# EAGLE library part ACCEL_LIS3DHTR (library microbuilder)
LIS3DHTR 3-Axis Accelerometer with I2C/SPI Interface VDD: 1.71-3.6V VDDIO: 1.71-VDD+0.1V Scale: +/-2g, 4g, 8g, 16g with 16--bit data output Temp:: -40°C - 85°C Mouser: 511-LIS3DHTR Digikey: 497-10613-1-ND
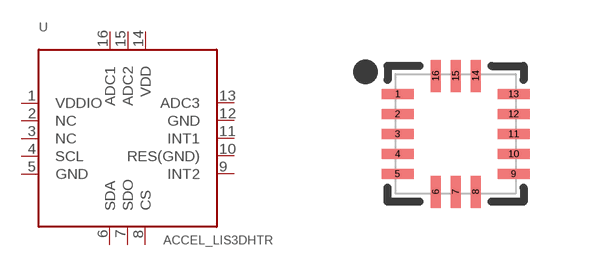
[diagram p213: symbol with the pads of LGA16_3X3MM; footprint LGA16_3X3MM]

Designator prefix U

## ACCEL_LIS3DHTR  [LGA16_3X3MM]
1  VDDIO  sup
2  NC  nc
3  NC  nc
4  SCL
5  GND  sup
6  SDA
7  SDO
8  CS  in
9  INT2  out
10  RES(GND)
11  INT1  out
12  GND  sup
13  ADC3  in
14  VDD  sup
15  ADC2  in
16  ADC1  in

## Footprint LGA16_3X3MM (pad centres in mm)
smd 0.8 x 0.25: 1 -1.45,1; 2 -1.45,0.5; 3 -1.45,0; 4 -1.45,-0.5; 5 -1.45,-1; 9 1.45,-1; 10 1.45,-0.5; 11 1.45,0; 12 1.45,0.5; 13 1.45,1
smd 0.25 x 0.8: 6 -0.5,-1.45; 7 0,-1.45; 8 0.5,-1.45; 14 0.5,1.45; 15 0,1.45; 16 -0.5,1.45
